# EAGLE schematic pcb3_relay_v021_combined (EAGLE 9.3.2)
Switching done with 30 x G6K-2F-Y 2xDPDT relays + 2 x HC-595

## Sheet 1 of 5: Amplitude & Frequency Detectors
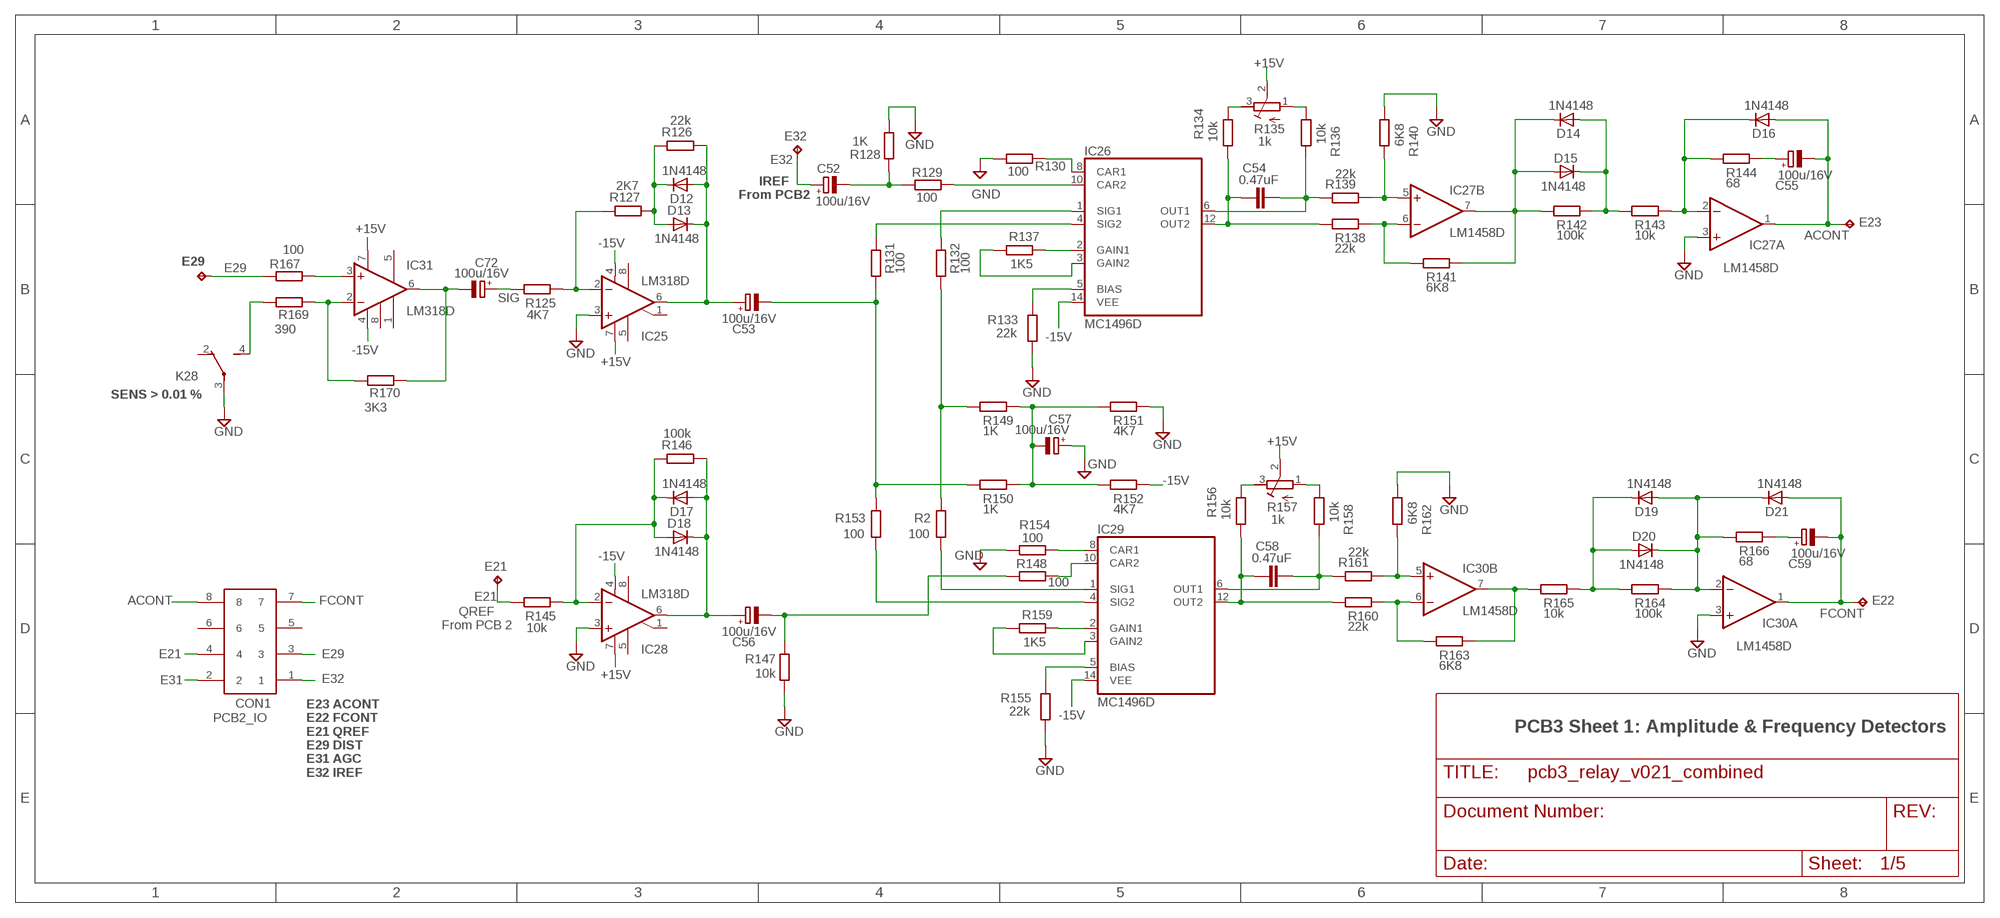
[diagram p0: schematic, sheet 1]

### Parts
C52  100u/16V  CPOL-EUUD-6,3X8,8  [UD-6,3X5,8_NICHICON]
C53  100u/16V  CPOL-EUUD-6,3X8,8  [UD-6,3X5,8_NICHICON]
C54  0.47uF  C-EUC1206  [C1206]
C55  100u/16V  CPOL-EUUD-6,3X8,8  [UD-6,3X5,8_NICHICON]
C56  100u/16V  CPOL-EUUD-6,3X8,8  [UD-6,3X5,8_NICHICON]
C57  100u/16V  CPOL-EUUD-6,3X8,8  [UD-6,3X5,8_NICHICON]
C58  0.47uF  C-EUC1206  [C1206]
C59  100u/16V  CPOL-EUUD-6,3X8,8  [UD-6,3X5,8_NICHICON]
C72  100u/16V  CPOL-EUUD-6,3X8,8  [UD-6,3X5,8_NICHICON]
CON1  PCB2_IO  61200821621  [61200821621]
D12  1N4148  D-SOD-80  [SOD80]
D13  1N4148  D-SOD-80  [SOD80]
D14  1N4148  D-SOD-80  [SOD80]
D15  1N4148  D-SOD-80  [SOD80]
D16  1N4148  D-SOD-80  [SOD80]
D17  1N4148  D-SOD-80  [SOD80]
D18  1N4148  D-SOD-80  [SOD80]
D19  1N4148  D-SOD-80  [SOD80]
D20  1N4148  D-SOD-80  [SOD80]
D21  1N4148  D-SOD-80  [SOD80]
E21  TPPAD1-13Y  [P1-13Y]
E22  TPPAD1-13Y  [P1-13Y]
E23  TPPAD1-13Y  [P1-13Y]
E29  TPPAD1-13Y  [P1-13Y]
E32  TPPAD1-13Y  [P1-13Y]
IC25  LM318D  [SO08]
IC26  MC1496D  [SOIC-14]
IC27  LM1458D  [SO08]
IC28  LM318D  [SO08]
IC29  MC1496D  [SOIC-14]
IC30  LM1458D  [SO08]
IC31  LM318D  [SOIC8]
K28  G6K-2F-Y  [G6K-2F-Y]
R2  100  R-EU_R1206  [R1206]
R125  4K7  R-EU_R1206  [R1206]
R126  22k  R-EU_R1206  [R1206]
R127  2K7  R-EU_R1206  [R1206]
R128  1K  R-EU_R1206  [R1206]
R129  100  R-EU_R1206  [R1206]
R130  100  R-EU_R1206  [R1206]
R131  100  R-EU_R1206  [R1206]
R132  100  R-EU_R1206  [R1206]
R133  22k  R-EU_R1206  [R1206]
R134  10k  R-EU_R1206  [R1206]
R135  1k  R-TRIMM3296W  [RTRIM3296W]
R136  10k  R-EU_R1206  [R1206]
R137  1K5  R-EU_R1206  [R1206]
R138  22k  R-EU_R1206  [R1206]
R139  22k  R-EU_R1206  [R1206]
R140  6K8  R-EU_R1206  [R1206]
R141  6K8  R-EU_R1206  [R1206]
R142  100k  R-EU_R1206  [R1206]
R143  10k  R-EU_R1206  [R1206]
R144  68  R-EU_R1206  [R1206]
R145  10k  R-EU_R1206  [R1206]
R146  100k  R-EU_R1206  [R1206]
R147  10k  R-EU_R1206  [R1206]
R148  100  R-EU_R1206  [R1206]
R149  1K  R-EU_R1206  [R1206]
R150  1K  R-EU_R1206  [R1206]
R151  4K7  R-EU_R1206  [R1206]
R152  4K7  R-EU_R1206  [R1206]
R153  100  R-EU_R1206  [R1206]
R154  100  R-EU_R1206  [R1206]
R155  22k  R-EU_R1206  [R1206]
R156  10k  R-EU_R1206  [R1206]
R157  1k  R-TRIMM3296W  [RTRIM3296W]
R158  10k  R-EU_R1206  [R1206]
R159  1K5  R-EU_R1206  [R1206]
R160  22k  R-EU_R1206  [R1206]
R161  22k  R-EU_R1206  [R1206]
R162  6K8  R-EU_R1206  [R1206]
R163  6K8  R-EU_R1206  [R1206]
R164  100k  R-EU_R1206  [R1206]
R165  10k  R-EU_R1206  [R1206]
R166  68  R-EU_R1206  [R1206]
R167  100  R-EU_R1206  [R1206]
R169  390  R-EU_R1206  [R1206]
R170  3K3  R-EU_R1206  [R1206]

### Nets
+15V: IC25.7(V+) IC28.7(V+) IC31.7(V+) R135.2(S) R157.2(S) ; also sheet 2,4,5
-15V: IC25.4(V-) IC26.14(VEE) IC28.4(V-) IC29.14(VEE) IC31.4(V-) R152.1 ; also sheet 2,4,5
ACONT: C55.- CON1.8 D16.2(A) E23.TP IC27.1(A:OUT)
E21: CON1.4 E21.TP R145.2
E29: CON1.3 E29.TP R167.1 ; also sheet 4
E31: CON1.2 ; also sheet 2
E32: C52.+ CON1.1 E32.TP
FCONT: C59.- CON1.7 D21.2(A) E22.TP IC30.1(A:OUT) ; also sheet 2
GND: C57.+ IC25.3(+IN) IC27.3(A:+IN) IC28.3(+IN) IC30.3(A:+IN) K28.3(2:P) R128.2 R130.2 R133.2 R140.2 R147.2 R151.1 R154.2 R155.2 R162.2 ; also sheet 2,3,4,5
N$1: IC26.8(CAR1) R130.1
N$17: IC25.2(-IN) R125.1 R127.1
N$22: D12.1(C) D13.2(A) R126.1 R127.2
N$24: C53.+ D12.2(A) D13.1(C) IC25.6(OUT) R126.2
N$27: D17.1(C) D18.2(A) IC28.2(-IN) R145.1 R146.1
N$28: C56.- R147.1 R148.2
N$29: C56.+ D17.2(A) D18.1(C) IC28.6(OUT) R146.2
N$30: IC26.3(GAIN2) R137.2
N$31: IC26.10(CAR2) R129.1
N$35: IC29.2(GAIN1) R159.1
N$36: R134.1 R135.3(E)
N$37: IC26.2(GAIN1) R137.1
N$38: IC26.5(BIAS) R133.1
N$39: IC29.5(BIAS) R155.1
N$40: IC29.8(CAR1) R154.1
N$41: IC26.4(SIG2) R131.1
N$42: IC26.1(SIG1) R132.1
N$43: C52.- R128.1 R129.2
N$44: C58.1 IC29.12(OUT2) R156.2 R160.2
N$45: C54.2 IC26.6(OUT1) R136.1 R139.1
N$46: C54.1 IC26.12(OUT2) R134.2 R138.2
N$47: IC27.5(B:+IN) R139.2 R140.1
N$48: IC27.6(B:-IN) R138.1 R141.2
N$49: IC29.10(CAR2) R148.1
N$50: D14.1(C) D15.2(A) IC27.7(B:OUT) R141.1 R142.2
N$51: D14.2(A) D15.1(C) R142.1 R143.2
N$52: D16.1(C) IC27.2(A:-IN) R143.1 R144.2
N$53: C55.+ R144.1
N$54: C53.- R131.2 R150.2 R153.1
N$55: R135.1(A) R136.2
N$56: IC29.4(SIG2) R153.2
N$57: IC29.3(GAIN2) R159.2
N$58: R156.1 R157.3(E)
N$59: R157.1(A) R158.2
N$60: C58.2 IC29.6(OUT1) R158.1 R161.1
N$61: IC30.5(B:+IN) R161.2 R162.1
N$62: IC30.6(B:-IN) R160.1 R163.2
N$63: D19.1(C) D20.2(A) R164.2 R165.1
N$64: D19.2(A) D20.1(C) D21.1(C) IC30.2(A:-IN) R164.1 R166.2
N$65: C72.- IC31.6(OUT) R170.1
N$66: C59.+ R166.1
N$67: IC29.1(SIG1) R2.2
N$68: R2.1 R132.2 R149.2
N$69: C57.- R149.1 R150.1 R151.2 R152.2
N$70: IC30.7(B:OUT) R163.1 R165.2
N$71: IC31.3(+IN) R167.2
N$72: K28.4(2:S) R169.2
N$73: IC31.2(-IN) R169.1 R170.2
SIG: C72.+ R125.2
Unconnected: CON1.5 CON1.6 IC25.1(ON/CMP) IC25.5(ON) IC25.8(CMP) IC28.1(ON/CMP) IC28.5(ON) IC28.8(CMP) IC31.1(BAL1) IC31.5(BAL2) IC31.8(COMP) K28.2(2:O)

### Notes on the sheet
- IREF
  From PCB2
- SENS > 0.01 %
- QREF
  From PCB 2
- PCB3 Sheet 1: Amplitude & Frequency Detectors
- E23 ACONT
  E22 FCONT
  E21 QREF
  E29 DIST
  E31 AGC
  E32 IREF

## Sheet 2 of 5: Meter + LEDs
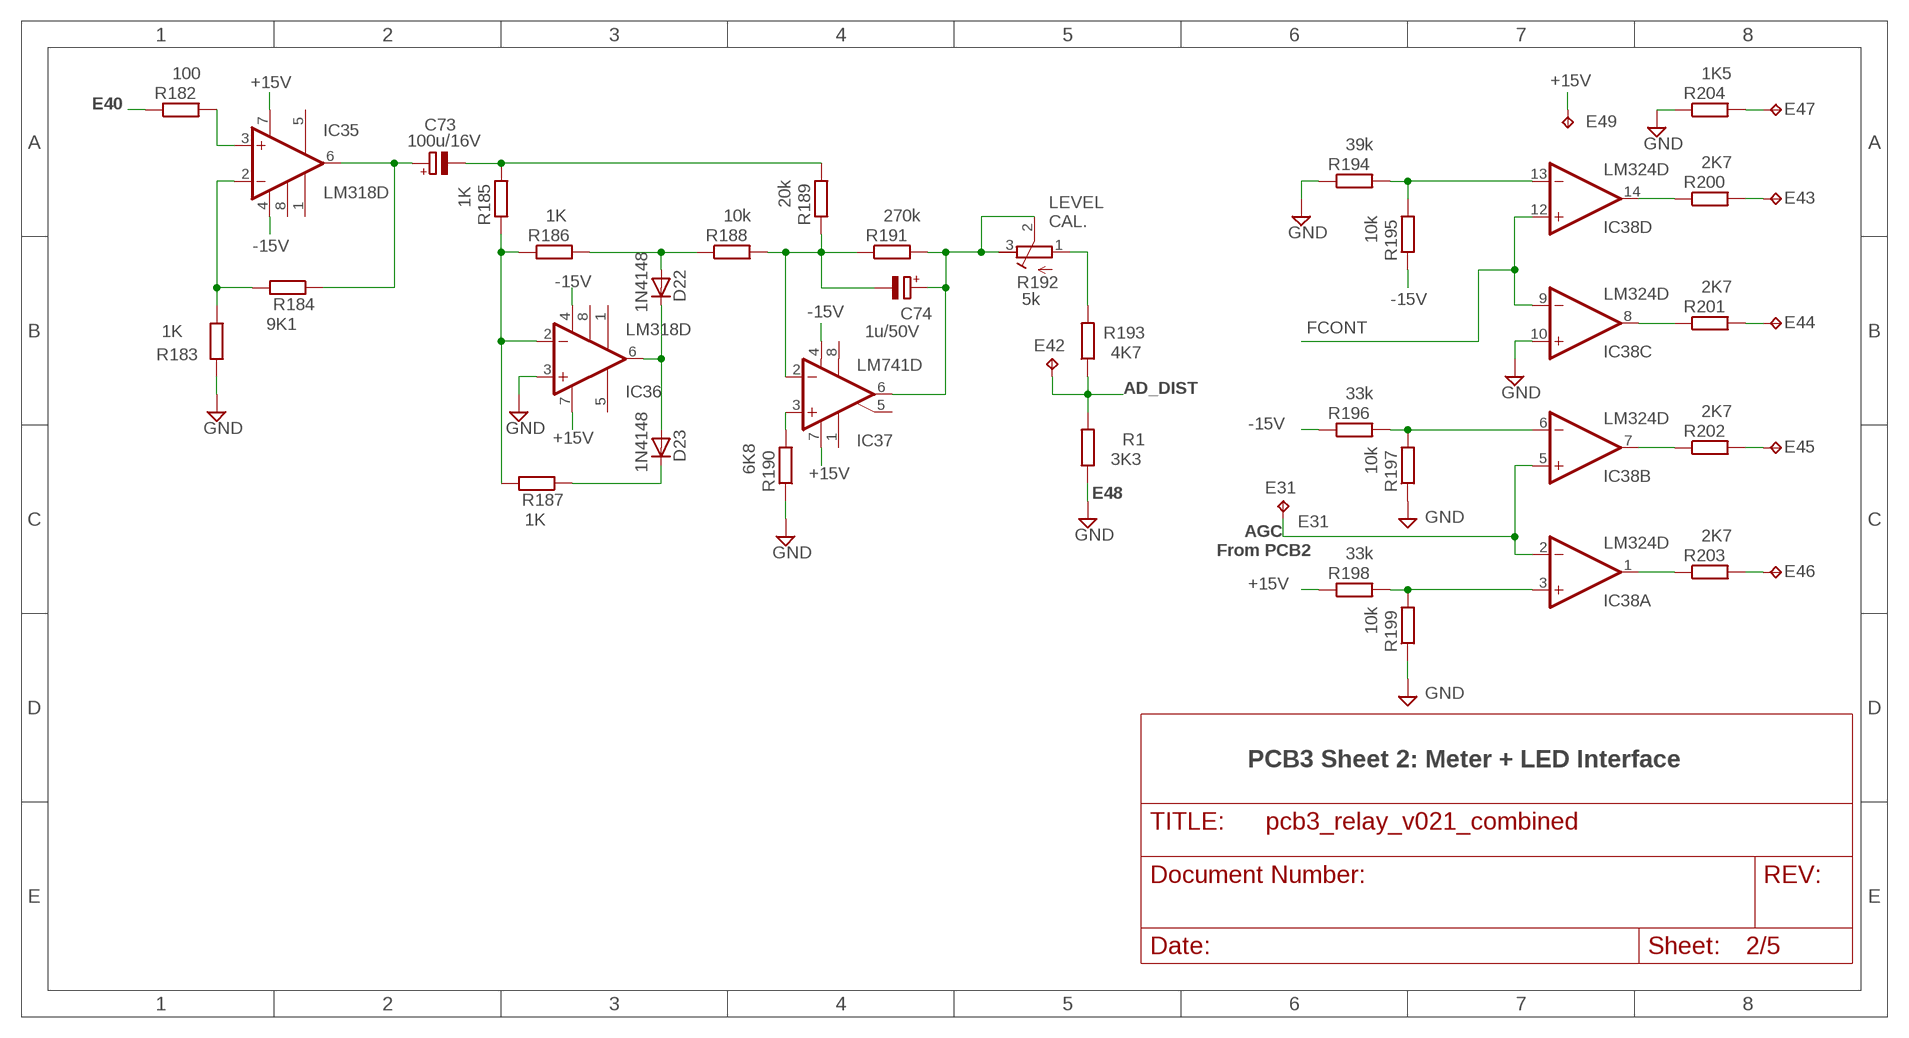
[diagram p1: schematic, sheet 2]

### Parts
C73  100u/16V  CPOL-EUUD-6,3X8,8  [UD-6,3X5,8_NICHICON]
C74  1u/50V  CPOL-EUUD-4X5,8  [UD-4X5,8_NICHICON]
D22  1N4148  D-SOD-80  [SOD80]
D23  1N4148  D-SOD-80  [SOD80]
E31  TPPAD1-13Y  [P1-13Y]
E42  TPPAD1-13Y  [P1-13Y]
E43  TPPAD1-13Y  [P1-13Y]
E44  TPPAD1-13Y  [P1-13Y]
E45  TPPAD1-13Y  [P1-13Y]
E46  TPPAD1-13Y  [P1-13Y]
E47  TPPAD1-13Y  [P1-13Y]
E49  TPPAD1-13Y  [P1-13Y]
IC35  LM318D  [SOIC8]
IC36  LM318D  [SOIC8]
IC37  LM741D  [SO08]
IC38  LM324D  [SO14]
R1  3K3  R-EU_R1206  [R1206]
R182  100  R-EU_R1206  [R1206]
R183  1K  R-EU_R1206  [R1206]
R184  9K1  R-EU_R1206  [R1206]
R185  1K  R-EU_R1206  [R1206]
R186  1K  R-EU_R1206  [R1206]
R187  1K  R-EU_R1206  [R1206]
R188  10k  R-EU_R1206  [R1206]
R189  20k  R-EU_R1206  [R1206]
R190  6K8  R-EU_R1206  [R1206]
R191  270k  R-EU_R1206  [R1206]
R192  5k  R-TRIMM3296W  [RTRIM3296W]
R193  4K7  R-EU_R1206  [R1206]
R194  39k  R-EU_R1206  [R1206]
R195  10k  R-EU_R1206  [R1206]
R196  33k  R-EU_R1206  [R1206]
R197  10k  R-EU_R1206  [R1206]
R198  33k  R-EU_R1206  [R1206]
R199  10k  R-EU_R1206  [R1206]
R200  2K7  R-EU_R1206  [R1206]
R201  2K7  R-EU_R1206  [R1206]
R202  2K7  R-EU_R1206  [R1206]
R203  2K7  R-EU_R1206  [R1206]
R204  1K5  R-EU_R1206  [R1206]

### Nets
+15V: E49.TP IC35.7(V+) IC36.7(V+) IC37.7(V+) R198.1 ; also sheet 1,4,5
-15V: IC35.4(V-) IC36.4(V-) IC37.4(V-) R195.1 R196.1 ; also sheet 1,4,5
AD_DIST: E42.TP R1.2 R193.1 ; also sheet 3
E31: E31.TP IC38.2(A:-IN) IC38.5(B:+IN) ; also sheet 1
E40: R182.1 ; also sheet 4
E43: E43.TP R200.2
E44: E44.TP R201.2
E45: E45.TP R202.2
E46: E46.TP R203.2
FCONT: IC38.9(C:-IN) IC38.12(D:+IN) ; also sheet 1
GND: IC36.3(+IN) IC38.10(C:+IN) R1.1 R183.2 R190.1 R194.1 R197.1 R199.1 R204.1 ; also sheet 1,3,4,5
N$2: R192.1(A) R193.2
N$3: IC37.3(+IN) R190.2
N$4: IC36.2(-IN) R185.1 R186.1 R187.2
N$5: D23.1(C) R187.1
N$6: D22.1(C) D23.2(A) IC36.6(OUT)
N$7: D22.2(A) R186.2 R188.1
N$8: C74.- IC37.2(-IN) R188.2 R189.1 R191.1
N$9: C74.+ IC37.6(OUT) R191.2 R192.2(S) R192.3(E)
N$10: C73.- R185.2 R189.2
N$11: IC38.13(D:-IN) R194.2 R195.2
N$12: IC38.3(A:+IN) R198.2 R199.2
N$13: IC38.6(B:-IN) R196.2 R197.2
N$14: IC38.1(A:OUT) R203.1
N$15: E47.TP R204.2
N$16: IC35.2(-IN) R183.1 R184.2
N$18: IC38.7(B:OUT) R202.1
N$19: IC38.8(C:OUT) R201.1
N$25: IC38.14(D:OUT) R200.1
N$81: IC35.3(+IN) R182.2
N$84: C73.+ IC35.6(OUT) R184.1
Unconnected: IC35.1(BAL1) IC35.5(BAL2) IC35.8(COMP) IC36.1(BAL1) IC36.5(BAL2) IC36.8(COMP) IC37.1(ON1) IC37.5(ON2) IC37.8(OPT)

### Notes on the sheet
- LEVEL
  CAL.
- E48
- AGC
  From PCB2
- PCB3 Sheet 2: Meter + LED Interface

## Sheet 3 of 5: Relays + Digital
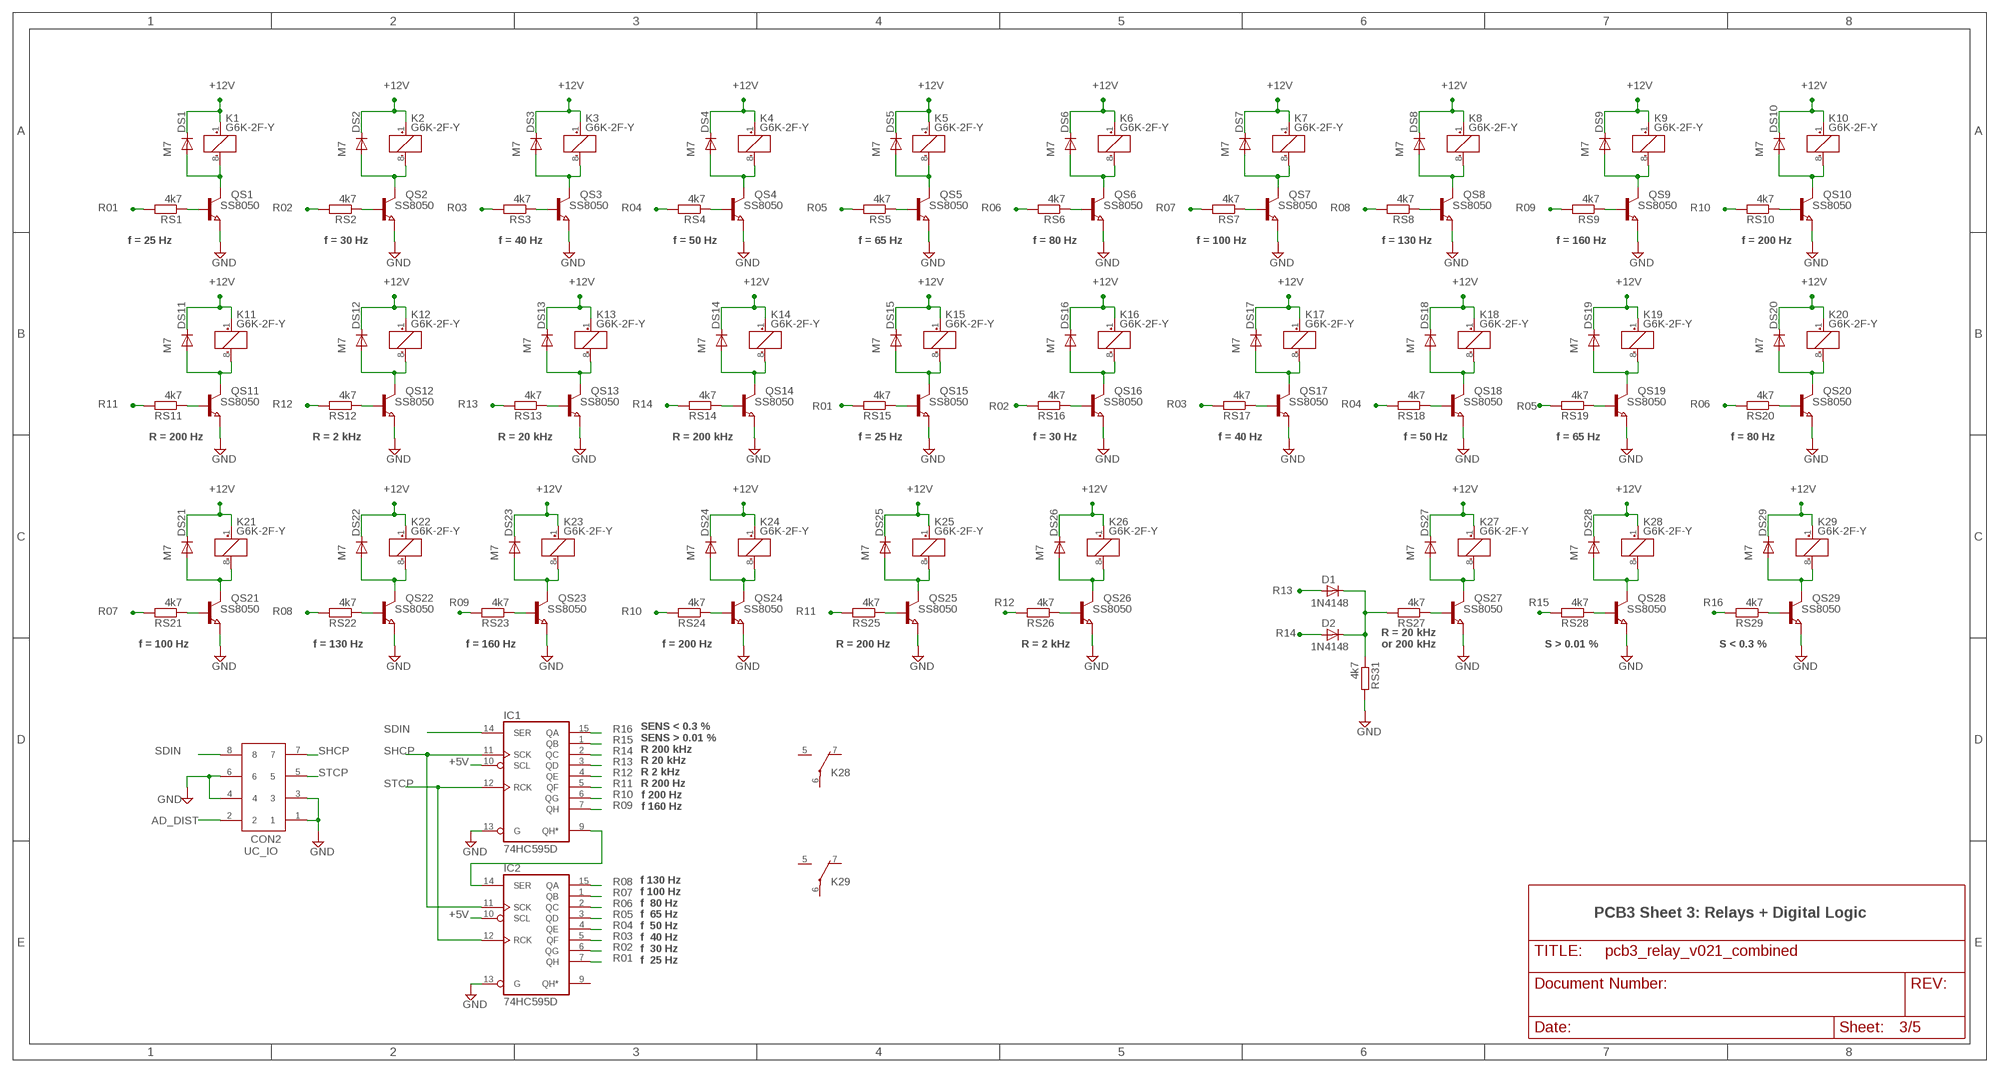
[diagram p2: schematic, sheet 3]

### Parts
CON2  UC_IO  61200821621  [61200821621]
D1  1N4148  D-SOD-80  [SOD80]
D2  1N4148  D-SOD-80  [SOD80]
DS1  M7  DIODE-DO214AC  [DO214AC]
DS2  M7  DIODE-DO214AC  [DO214AC]
DS3  M7  DIODE-DO214AC  [DO214AC]
DS4  M7  DIODE-DO214AC  [DO214AC]
DS5  M7  DIODE-DO214AC  [DO214AC]
DS6  M7  DIODE-DO214AC  [DO214AC]
DS7  M7  DIODE-DO214AC  [DO214AC]
DS8  M7  DIODE-DO214AC  [DO214AC]
DS9  M7  DIODE-DO214AC  [DO214AC]
DS10  M7  DIODE-DO214AC  [DO214AC]
DS11  M7  DIODE-DO214AC  [DO214AC]
DS12  M7  DIODE-DO214AC  [DO214AC]
DS13  M7  DIODE-DO214AC  [DO214AC]
DS14  M7  DIODE-DO214AC  [DO214AC]
DS15  M7  DIODE-DO214AC  [DO214AC]
DS16  M7  DIODE-DO214AC  [DO214AC]
DS17  M7  DIODE-DO214AC  [DO214AC]
DS18  M7  DIODE-DO214AC  [DO214AC]
DS19  M7  DIODE-DO214AC  [DO214AC]
DS20  M7  DIODE-DO214AC  [DO214AC]
DS21  M7  DIODE-DO214AC  [DO214AC]
DS22  M7  DIODE-DO214AC  [DO214AC]
DS23  M7  DIODE-DO214AC  [DO214AC]
DS24  M7  DIODE-DO214AC  [DO214AC]
DS25  M7  DIODE-DO214AC  [DO214AC]
DS26  M7  DIODE-DO214AC  [DO214AC]
DS27  M7  DIODE-DO214AC  [DO214AC]
DS28  M7  DIODE-DO214AC  [DO214AC]
DS29  M7  DIODE-DO214AC  [DO214AC]
IC1  74HC595D  [SO16]
IC2  74HC595D  [SO16]
K1  G6K-2F-Y  [G6K-2F-Y]
K2  G6K-2F-Y  [G6K-2F-Y]
K3  G6K-2F-Y  [G6K-2F-Y]
K4  G6K-2F-Y  [G6K-2F-Y]
K5  G6K-2F-Y  [G6K-2F-Y]
K6  G6K-2F-Y  [G6K-2F-Y]
K7  G6K-2F-Y  [G6K-2F-Y]
K8  G6K-2F-Y  [G6K-2F-Y]
K9  G6K-2F-Y  [G6K-2F-Y]
K10  G6K-2F-Y  [G6K-2F-Y]
K11  G6K-2F-Y  [G6K-2F-Y]
K12  G6K-2F-Y  [G6K-2F-Y]
K13  G6K-2F-Y  [G6K-2F-Y]
K14  G6K-2F-Y  [G6K-2F-Y]
K15  G6K-2F-Y  [G6K-2F-Y]
K16  G6K-2F-Y  [G6K-2F-Y]
K17  G6K-2F-Y  [G6K-2F-Y]
K18  G6K-2F-Y  [G6K-2F-Y]
K19  G6K-2F-Y  [G6K-2F-Y]
K20  G6K-2F-Y  [G6K-2F-Y]
K21  G6K-2F-Y  [G6K-2F-Y]
K22  G6K-2F-Y  [G6K-2F-Y]
K23  G6K-2F-Y  [G6K-2F-Y]
K24  G6K-2F-Y  [G6K-2F-Y]
K25  G6K-2F-Y  [G6K-2F-Y]
K26  G6K-2F-Y  [G6K-2F-Y]
K27  G6K-2F-Y  [G6K-2F-Y]
K29  G6K-2F-Y  [G6K-2F-Y]
QS1  SS8050  NPN-TRANSISTOR_SOT23  [SOT23]
QS2  SS8050  NPN-TRANSISTOR_SOT23  [SOT23]
QS3  SS8050  NPN-TRANSISTOR_SOT23  [SOT23]
QS4  SS8050  NPN-TRANSISTOR_SOT23  [SOT23]
QS5  SS8050  NPN-TRANSISTOR_SOT23  [SOT23]
QS6  SS8050  NPN-TRANSISTOR_SOT23  [SOT23]
QS7  SS8050  NPN-TRANSISTOR_SOT23  [SOT23]
QS8  SS8050  NPN-TRANSISTOR_SOT23  [SOT23]
QS9  SS8050  NPN-TRANSISTOR_SOT23  [SOT23]
QS10  SS8050  NPN-TRANSISTOR_SOT23  [SOT23]
QS11  SS8050  NPN-TRANSISTOR_SOT23  [SOT23]
QS12  SS8050  NPN-TRANSISTOR_SOT23  [SOT23]
QS13  SS8050  NPN-TRANSISTOR_SOT23  [SOT23]
QS14  SS8050  NPN-TRANSISTOR_SOT23  [SOT23]
QS15  SS8050  NPN-TRANSISTOR_SOT23  [SOT23]
QS16  SS8050  NPN-TRANSISTOR_SOT23  [SOT23]
QS17  SS8050  NPN-TRANSISTOR_SOT23  [SOT23]
QS18  SS8050  NPN-TRANSISTOR_SOT23  [SOT23]
QS19  SS8050  NPN-TRANSISTOR_SOT23  [SOT23]
QS20  SS8050  NPN-TRANSISTOR_SOT23  [SOT23]
QS21  SS8050  NPN-TRANSISTOR_SOT23  [SOT23]
QS22  SS8050  NPN-TRANSISTOR_SOT23  [SOT23]
QS23  SS8050  NPN-TRANSISTOR_SOT23  [SOT23]
QS24  SS8050  NPN-TRANSISTOR_SOT23  [SOT23]
QS25  SS8050  NPN-TRANSISTOR_SOT23  [SOT23]
QS26  SS8050  NPN-TRANSISTOR_SOT23  [SOT23]
QS27  SS8050  NPN-TRANSISTOR_SOT23  [SOT23]
QS28  SS8050  NPN-TRANSISTOR_SOT23  [SOT23]
QS29  SS8050  NPN-TRANSISTOR_SOT23  [SOT23]
RS1  4k7  R-EU_M1206  [M1206]
RS2  4k7  R-EU_M1206  [M1206]
RS3  4k7  R-EU_M1206  [M1206]
RS4  4k7  R-EU_M1206  [M1206]
RS5  4k7  R-EU_M1206  [M1206]
RS6  4k7  R-EU_M1206  [M1206]
RS7  4k7  R-EU_M1206  [M1206]
RS8  4k7  R-EU_M1206  [M1206]
RS9  4k7  R-EU_M1206  [M1206]
RS10  4k7  R-EU_M1206  [M1206]
RS11  4k7  R-EU_M1206  [M1206]
RS12  4k7  R-EU_M1206  [M1206]
RS13  4k7  R-EU_M1206  [M1206]
RS14  4k7  R-EU_M1206  [M1206]
RS15  4k7  R-EU_M1206  [M1206]
RS16  4k7  R-EU_M1206  [M1206]
RS17  4k7  R-EU_M1206  [M1206]
RS18  4k7  R-EU_M1206  [M1206]
RS19  4k7  R-EU_M1206  [M1206]
RS20  4k7  R-EU_M1206  [M1206]
RS21  4k7  R-EU_M1206  [M1206]
RS22  4k7  R-EU_M1206  [M1206]
RS23  4k7  R-EU_M1206  [M1206]
RS24  4k7  R-EU_M1206  [M1206]
RS25  4k7  R-EU_M1206  [M1206]
RS26  4k7  R-EU_M1206  [M1206]
RS27  4k7  R-EU_M1206  [M1206]
RS28  4k7  R-EU_M1206  [M1206]
RS29  4k7  R-EU_M1206  [M1206]
RS31  4k7  R-EU_M1206  [M1206]

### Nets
+5V: IC1.10(SCL) IC2.10(SCL) ; also sheet 5
+12V: DS1.C DS2.C DS3.C DS4.C DS5.C DS6.C DS7.C DS8.C DS9.C DS10.C DS11.C DS12.C DS13.C DS14.C DS15.C DS16.C DS17.C DS18.C DS19.C DS20.C DS21.C DS22.C DS23.C DS24.C DS25.C DS26.C DS27.C DS28.C DS29.C K1.1(1:+) K2.1(1:+) K3.1(1:+) K4.1(1:+) K5.1(1:+) K6.1(1:+) K7.1(1:+) K8.1(1:+) K9.1(1:+) K10.1(1:+) K11.1(1:+) K12.1(1:+) K13.1(1:+) K14.1(1:+) K15.1(1:+) K16.1(1:+) K17.1(1:+) K18.1(1:+) K19.1(1:+) K20.1(1:+) K21.1(1:+) K22.1(1:+) K23.1(1:+) K24.1(1:+) K25.1(1:+) K26.1(1:+) K27.1(1:+) K28.1(1:+) K29.1(1:+) ; also sheet 5
AD_DIST: CON2.2 ; also sheet 2
GND: CON2.1 CON2.3 CON2.4 CON2.6 IC1.13(G) IC2.13(G) QS1.2(E) QS2.2(E) QS3.2(E) QS4.2(E) QS5.2(E) QS6.2(E) QS7.2(E) QS8.2(E) QS9.2(E) QS10.2(E) QS11.2(E) QS12.2(E) QS13.2(E) QS14.2(E) QS15.2(E) QS16.2(E) QS17.2(E) QS18.2(E) QS19.2(E) QS20.2(E) QS21.2(E) QS22.2(E) QS23.2(E) QS24.2(E) QS25.2(E) QS26.2(E) QS27.2(E) QS28.2(E) QS29.2(E) RS31.2 ; also sheet 1,2,4,5
N$74: D1.1(C) D2.1(C) RS27.2 RS31.1
N$101: QS1.1(B) RS1.1
N$102: DS1.A K1.8(1:-) QS1.3(C)
N$103: QS2.1(B) RS2.1
N$104: DS2.A K2.8(1:-) QS2.3(C)
N$105: QS3.1(B) RS3.1
N$106: DS3.A K3.8(1:-) QS3.3(C)
N$107: QS4.1(B) RS4.1
N$108: DS4.A K4.8(1:-) QS4.3(C)
N$109: QS5.1(B) RS5.1
N$110: DS5.A K5.8(1:-) QS5.3(C)
N$111: QS6.1(B) RS6.1
N$112: DS6.A K6.8(1:-) QS6.3(C)
N$113: QS7.1(B) RS7.1
N$114: DS7.A K7.8(1:-) QS7.3(C)
N$115: QS8.1(B) RS8.1
N$116: DS8.A K8.8(1:-) QS8.3(C)
N$117: QS9.1(B) RS9.1
N$118: DS9.A K9.8(1:-) QS9.3(C)
N$119: QS10.1(B) RS10.1
N$120: DS10.A K10.8(1:-) QS10.3(C)
N$124: QS11.1(B) RS11.1
N$125: DS11.A K11.8(1:-) QS11.3(C)
N$126: QS12.1(B) RS12.1
N$127: DS12.A K12.8(1:-) QS12.3(C)
N$128: QS13.1(B) RS13.1
N$129: DS13.A K13.8(1:-) QS13.3(C)
N$130: QS14.1(B) RS14.1
N$131: DS14.A K14.8(1:-) QS14.3(C)
N$132: QS16.1(B) RS16.1
N$133: DS16.A K16.8(1:-) QS16.3(C)
N$134: QS17.1(B) RS17.1
N$135: DS17.A K17.8(1:-) QS17.3(C)
N$136: QS18.1(B) RS18.1
N$137: DS18.A K18.8(1:-) QS18.3(C)
N$138: QS23.1(B) RS23.1
N$139: DS23.A K23.8(1:-) QS23.3(C)
N$140: QS19.1(B) RS19.1
N$141: DS19.A K19.8(1:-) QS19.3(C)
N$142: QS20.1(B) RS20.1
N$143: DS20.A K20.8(1:-) QS20.3(C)
N$144: QS21.1(B) RS21.1
N$145: DS21.A K21.8(1:-) QS21.3(C)
N$146: QS22.1(B) RS22.1
N$147: DS22.A K22.8(1:-) QS22.3(C)
N$148: QS15.1(B) RS15.1
N$149: DS15.A K15.8(1:-) QS15.3(C)
N$151: IC1.9(QH*) IC2.14(SER)
N$183: QS27.1(B) RS27.1
N$184: DS27.A K27.8(1:-) QS27.3(C)
N$185: QS24.1(B) RS24.1
N$186: DS24.A K24.8(1:-) QS24.3(C)
N$187: QS25.1(B) RS25.1
N$188: DS25.A K25.8(1:-) QS25.3(C)
N$189: QS26.1(B) RS26.1
N$190: DS26.A K26.8(1:-) QS26.3(C)
N$193: QS28.1(B) RS28.1
N$194: DS28.A K28.8(1:-) QS28.3(C)
N$195: QS29.1(B) RS29.1
N$196: DS29.A K29.8(1:-) QS29.3(C)
R01: IC2.7(QH) RS1.2 RS15.2
R02: IC2.6(QG) RS2.2 RS16.2
R03: IC2.5(QF) RS3.2 RS17.2
R04: IC2.4(QE) RS4.2 RS18.2
R05: IC2.3(QD) RS5.2 RS19.2
R06: IC2.2(QC) RS6.2 RS20.2
R07: IC2.1(QB) RS7.2 RS21.2
R08: IC2.15(QA) RS8.2 RS22.2
R09: IC1.7(QH) RS9.2 RS23.2
R10: IC1.6(QG) RS10.2 RS24.2
R11: IC1.5(QF) RS11.2 RS25.2
R12: IC1.4(QE) RS12.2 RS26.2
R13: D1.2(A) IC1.3(QD) RS13.2
R14: D2.2(A) IC1.2(QC) RS14.2
R15: IC1.1(QB) RS28.2
R16: IC1.15(QA) RS29.2
SDIN: CON2.8 IC1.14(SER)
SHCP: CON2.7 IC1.11(SCK) IC2.11(SCK)
STCP: CON2.5 IC1.12(RCK) IC2.12(RCK)
Unconnected: IC2.9(QH*) K28.5(3:S) K28.6(3:P) K28.7(3:O) K29.5(3:S) K29.6(3:P) K29.7(3:O)

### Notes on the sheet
- f = 25 Hz | f = 30 Hz | f = 40 Hz | f = 50 Hz | f = 65 Hz | f = 80 Hz | f = 100 Hz | f = 130 Hz | f = 160 Hz | f = 200 Hz
- R = 200 Hz | R = 2 kHz | R = 20 kHz | R = 200 kHz | f = 25 Hz | f = 30 Hz | f = 40 Hz | f = 50 Hz | f = 65 Hz | f = 80 Hz
- f = 100 Hz | f = 130 Hz | f = 160 Hz | f = 200 Hz | R = 200 Hz | R = 2 kHz
- R = 20 kHz
  or 200 kHz
- S > 0.01 % | S < 0.3 %
- SENS < 0.3 %
  SENS > 0.01 %
  R 200 kHz
  R 20 kHz
  R 2 kHz
  R 200 Hz
  f 200 Hz
  f 160 Hz
- PCB3 Sheet 3: Relays + Digital Logic
- f 130 Hz
  f 100 Hz
  f  80 Hz
  f  65 Hz
  f  50 Hz
  f  40 Hz
  f  30 Hz
  f  25 Hz

## Sheet 4 of 5: Filter Circuit
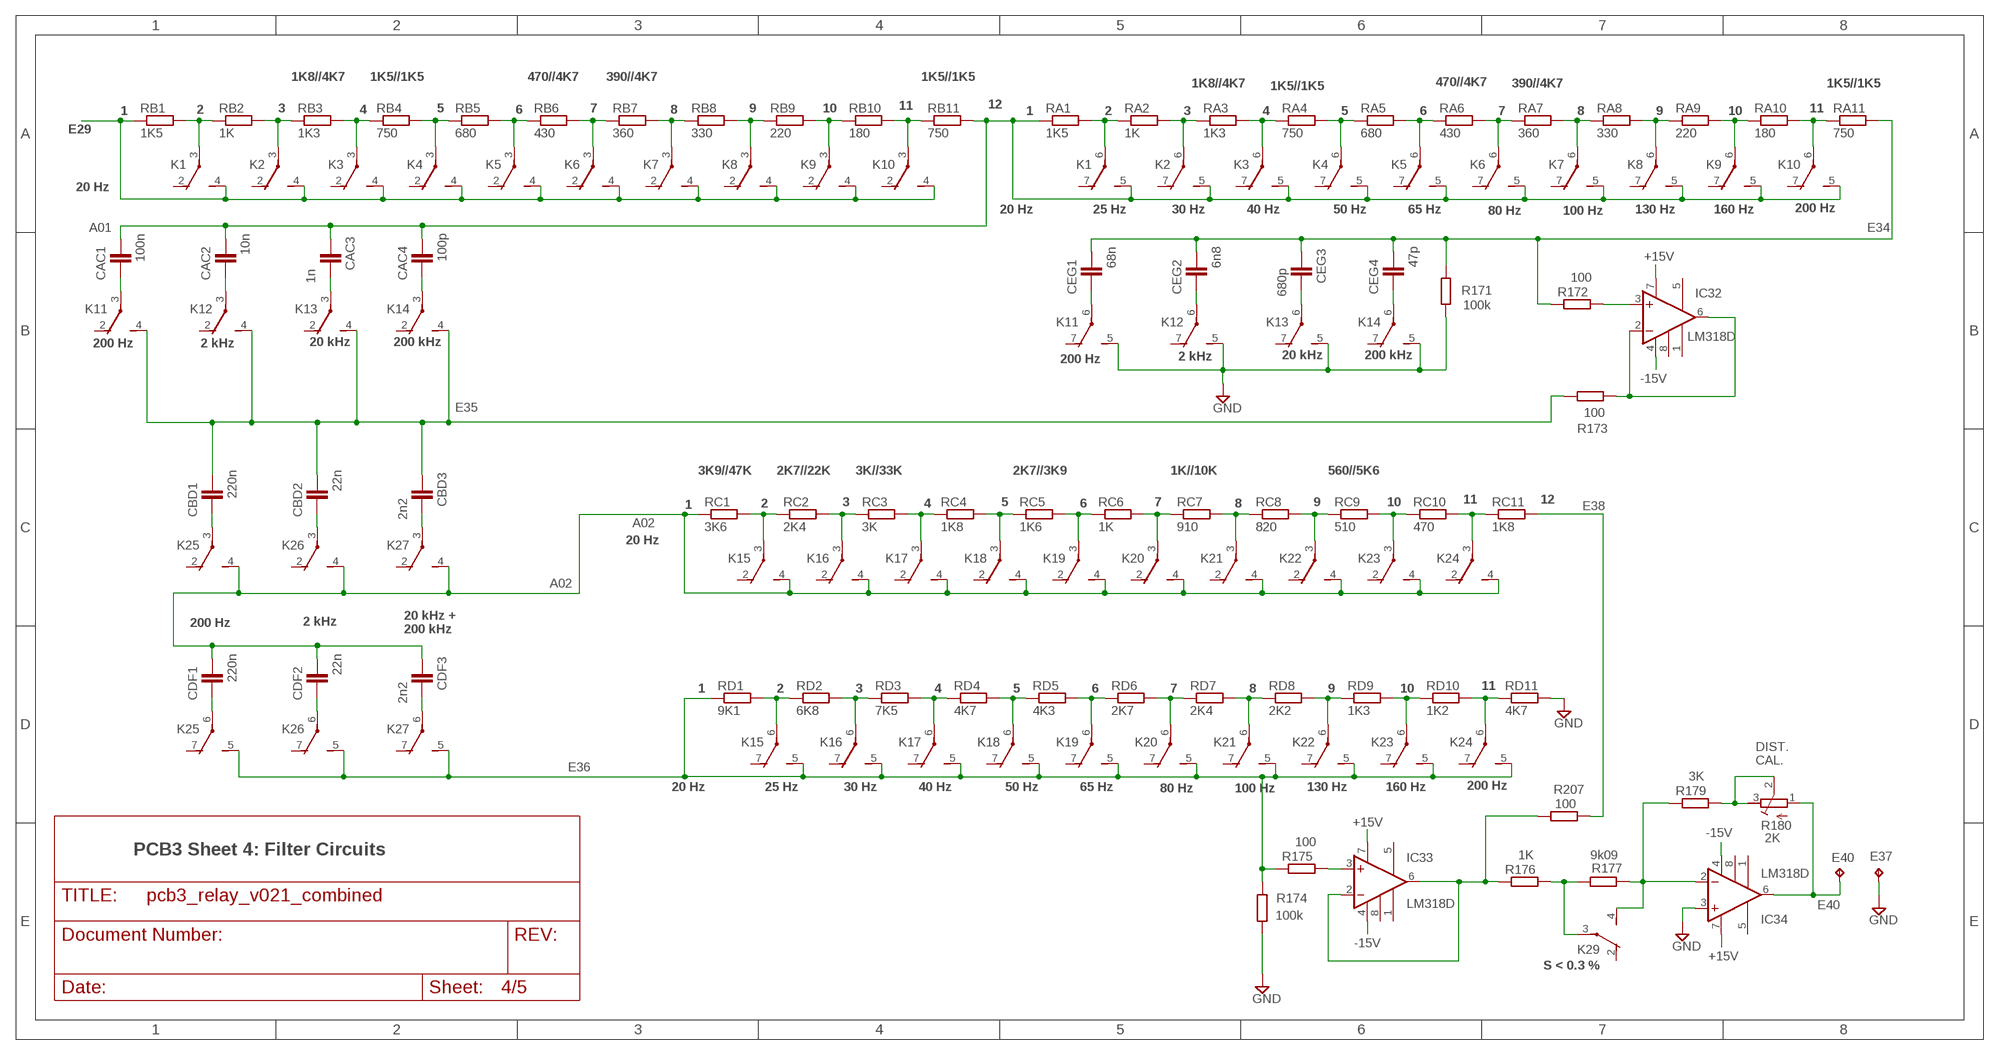
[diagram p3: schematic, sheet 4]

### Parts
CAC1  100n  C-EUC1206  [C1206]
CAC2  10n  C-EUC1206  [C1206]
CAC3  1n  C-EUC1206  [C1206]
CAC4  100p  C-EUC1206  [C1206]
CBD1  220n  C-EUC1206  [C1206]
CBD2  22n  C-EUC1206  [C1206]
CBD3  2n2  C-EUC1206  [C1206]
CDF1  220n  C-EUC1206  [C1206]
CDF2  22n  C-EUC1206  [C1206]
CDF3  2n2  C-EUC1206  [C1206]
CEG1  68n  C-EUC1206  [C1206]
CEG2  6n8  C-EUC1206  [C1206]
CEG3  680p  C-EUC1206  [C1206]
CEG4  47p  C-EUC1206  [C1206]
E37  TPPAD1-13Y  [P1-13Y]
E40  TPPAD1-13Y  [P1-13Y]
IC32  LM318D  [SOIC8]
IC33  LM318D  [SOIC8]
IC34  LM318D  [SOIC8]
R171  100k  R-EU_R1206  [R1206]
R172  100  R-EU_R1206  [R1206]
R173  100  R-EU_R1206  [R1206]
R174  100k  R-EU_R1206  [R1206]
R175  100  R-EU_R1206  [R1206]
R176  1K  R-EU_R1206  [R1206]
R177  9k09  R-EU_R1206  [R1206]
R179  3K  R-EU_R1206  [R1206]
R180  2K  R-TRIMM3296W  [RTRIM3296W]
R207  100  R-EU_R1206  [R1206]
RA1  1K5  R-EU_R1206  [R1206]
RA2  1K  R-EU_R1206  [R1206]
RA3  1K3  R-EU_R1206  [R1206]
RA4  750  R-EU_R1206  [R1206]
RA5  680  R-EU_R1206  [R1206]
RA6  430  R-EU_R1206  [R1206]
RA7  360  R-EU_R1206  [R1206]
RA8  330  R-EU_R1206  [R1206]
RA9  220  R-EU_R1206  [R1206]
RA10  180  R-EU_R1206  [R1206]
RA11  750  R-EU_R1206  [R1206]
RB1  1K5  R-EU_R1206  [R1206]
RB2  1K  R-EU_R1206  [R1206]
RB3  1K3  R-EU_R1206  [R1206]
RB4  750  R-EU_R1206  [R1206]
RB5  680  R-EU_R1206  [R1206]
RB6  430  R-EU_R1206  [R1206]
RB7  360  R-EU_R1206  [R1206]
RB8  330  R-EU_R1206  [R1206]
RB9  220  R-EU_R1206  [R1206]
RB10  180  R-EU_R1206  [R1206]
RB11  750  R-EU_R1206  [R1206]
RC1  3K6  R-EU_R1206  [R1206]
RC2  2K4  R-EU_R1206  [R1206]
RC3  3K  R-EU_R1206  [R1206]
RC4  1K8  R-EU_R1206  [R1206]
RC5  1K6  R-EU_R1206  [R1206]
RC6  1K  R-EU_R1206  [R1206]
RC7  910  R-EU_R1206  [R1206]
RC8  820  R-EU_R1206  [R1206]
RC9  510  R-EU_R1206  [R1206]
RC10  470  R-EU_R1206  [R1206]
RC11  1K8  R-EU_R1206  [R1206]
RD1  9K1  R-EU_R1206  [R1206]
RD2  6K8  R-EU_R1206  [R1206]
RD3  7K5  R-EU_R1206  [R1206]
RD4  4K7  R-EU_R1206  [R1206]
RD5  4K3  R-EU_R1206  [R1206]
RD6  2K7  R-EU_R1206  [R1206]
RD7  2K4  R-EU_R1206  [R1206]
RD8  2K2  R-EU_R1206  [R1206]
RD9  1K3  R-EU_R1206  [R1206]
RD10  1K2  R-EU_R1206  [R1206]
RD11  4K7  R-EU_R1206  [R1206]

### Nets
+15V: IC32.7(V+) IC33.7(V+) IC34.7(V+) ; also sheet 1,2,5
-15V: IC32.4(V-) IC33.4(V-) IC34.4(V-) ; also sheet 1,2,5
A01: CAC1.2 CAC2.2 CAC3.1 CAC4.2 K1.5(3:S) K2.5(3:S) K3.5(3:S) K4.5(3:S) K5.5(3:S) K6.5(3:S) K7.5(3:S) K8.5(3:S) K9.5(3:S) K10.5(3:S) RA1.1 RB11.2
A02: CDF1.2 CDF2.2 CDF3.1 K15.4(2:S) K16.4(2:S) K17.4(2:S) K18.4(2:S) K19.4(2:S) K20.4(2:S) K21.4(2:S) K22.4(2:S) K23.4(2:S) K24.4(2:S) K25.4(2:S) K26.4(2:S) K27.4(2:S) RC1.1
E29: K1.4(2:S) K2.4(2:S) K3.4(2:S) K4.4(2:S) K5.4(2:S) K6.4(2:S) K7.4(2:S) K8.4(2:S) K9.4(2:S) K10.4(2:S) RB1.1 ; also sheet 1
E34: CEG1.2 CEG2.2 CEG3.1 CEG4.2 R171.2 R172.1 RA11.2
E35: CBD1.2 CBD2.2 CBD3.1 K11.4(2:S) K12.4(2:S) K13.4(2:S) K14.4(2:S) R173.2
E36: K15.5(3:S) K16.5(3:S) K17.5(3:S) K18.5(3:S) K19.5(3:S) K20.5(3:S) K21.5(3:S) K22.5(3:S) K23.5(3:S) K24.5(3:S) K25.5(3:S) K26.5(3:S) K27.5(3:S) R174.2 R175.1 RD1.1
E38: R207.1 RC11.2
E40: E40.TP IC34.6(OUT) R180.1(A) ; also sheet 2
GND: E37.TP IC34.3(+IN) K11.5(3:S) K12.5(3:S) K13.5(3:S) K14.5(3:S) R171.1 R174.1 RD11.2 ; also sheet 1,2,3,5
N$20: K1.3(2:P) RB1.2 RB2.1
N$21: R179.2 R180.2(S) R180.3(E)
N$23: K2.3(2:P) RB2.2 RB3.1
N$26: K3.3(2:P) RB3.2 RB4.1
N$32: K4.3(2:P) RB4.2 RB5.1
N$33: IC32.2(-IN) IC32.6(OUT) R173.1
N$34: IC32.3(+IN) R172.2
N$75: IC33.3(+IN) R175.2
N$76: IC33.2(-IN) IC33.6(OUT) R176.1 R207.2
N$79: K29.3(2:P) R176.2 R177.1
N$80: IC34.2(-IN) K29.4(2:S) R177.2 R179.1
N$85: K5.3(2:P) RB5.2 RB6.1
N$86: K6.3(2:P) RB6.2 RB7.1
N$87: K7.3(2:P) RB7.2 RB8.1
N$88: K8.3(2:P) RB8.2 RB9.1
N$89: K9.3(2:P) RB9.2 RB10.1
N$90: K10.3(2:P) RB10.2 RB11.1
N$91: K1.6(3:P) RA1.2 RA2.1
N$92: K2.6(3:P) RA2.2 RA3.1
N$93: K3.6(3:P) RA3.2 RA4.1
N$94: K4.6(3:P) RA4.2 RA5.1
N$95: K5.6(3:P) RA5.2 RA6.1
N$96: K6.6(3:P) RA6.2 RA7.1
N$97: K7.6(3:P) RA7.2 RA8.1
N$98: K8.6(3:P) RA8.2 RA9.1
N$99: K9.6(3:P) RA9.2 RA10.1
N$100: K10.6(3:P) RA10.2 RA11.1
N$121: CAC1.1 K11.3(2:P)
N$122: CAC2.1 K12.3(2:P)
N$123: CAC3.2 K13.3(2:P)
N$152: CEG1.1 K11.6(3:P)
N$153: CEG2.1 K12.6(3:P)
N$154: CEG3.2 K13.6(3:P)
N$155: CAC4.1 K14.3(2:P)
N$156: CEG4.1 K14.6(3:P)
N$157: K15.3(2:P) RC1.2 RC2.1
N$158: K16.3(2:P) RC2.2 RC3.1
N$159: K17.3(2:P) RC3.2 RC4.1
N$160: K18.3(2:P) RC4.2 RC5.1
N$161: K19.3(2:P) RC5.2 RC6.1
N$162: K20.3(2:P) RC6.2 RC7.1
N$163: K21.3(2:P) RC7.2 RC8.1
N$164: K22.3(2:P) RC8.2 RC9.1
N$165: K23.3(2:P) RC9.2 RC10.1
N$166: K24.3(2:P) RC10.2 RC11.1
N$167: K15.6(3:P) RD1.2 RD2.1
N$168: K16.6(3:P) RD2.2 RD3.1
N$169: K17.6(3:P) RD3.2 RD4.1
N$170: K18.6(3:P) RD4.2 RD5.1
N$171: K19.6(3:P) RD5.2 RD6.1
N$172: K20.6(3:P) RD6.2 RD7.1
N$173: K21.6(3:P) RD7.2 RD8.1
N$174: K22.6(3:P) RD8.2 RD9.1
N$175: K23.6(3:P) RD9.2 RD10.1
N$176: K24.6(3:P) RD10.2 RD11.1
N$177: CBD1.1 K25.3(2:P)
N$178: CBD2.1 K26.3(2:P)
N$179: CBD3.2 K27.3(2:P)
N$180: CDF1.1 K25.6(3:P)
N$181: CDF2.1 K26.6(3:P)
N$182: CDF3.2 K27.6(3:P)
Unconnected: IC32.1(BAL1) IC32.5(BAL2) IC32.8(COMP) IC33.1(BAL1) IC33.5(BAL2) IC33.8(COMP) IC34.1(BAL1) IC34.5(BAL2) IC34.8(COMP) K1.2(2:O) K1.7(3:O) K2.2(2:O) K2.7(3:O) K3.2(2:O) K3.7(3:O) K4.2(2:O) K4.7(3:O) K5.2(2:O) K5.7(3:O) K6.2(2:O) K6.7(3:O) K7.2(2:O) K7.7(3:O) K8.2(2:O) K8.7(3:O) K9.2(2:O) K9.7(3:O) K10.2(2:O) K10.7(3:O) K11.2(2:O) K11.7(3:O) K12.2(2:O) K12.7(3:O) K13.2(2:O) K13.7(3:O) K14.2(2:O) K14.7(3:O) K15.2(2:O) K15.7(3:O) K16.2(2:O) K16.7(3:O) K17.2(2:O) K17.7(3:O) K18.2(2:O) K18.7(3:O) K19.2(2:O) K19.7(3:O) K20.2(2:O) K20.7(3:O) K21.2(2:O) K21.7(3:O) K22.2(2:O) K22.7(3:O) K23.2(2:O) K23.7(3:O) K24.2(2:O) K24.7(3:O) K25.2(2:O) K25.7(3:O) K26.2(2:O) K26.7(3:O) K27.2(2:O) K27.7(3:O) K29.2(2:O)

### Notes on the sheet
- 1K8//4K7 | 1K5//1K5 | 470//4K7 | 390//4K7 | 1K5//1K5
- 1K8//4K7 | 470//4K7 | 390//4K7 | 1K5//1K5
- 1K5//1K5
- 11 | 12
- 1 | 2 | 3 | 4 | 5 | 6 | 7 | 8 | 9 | 10 | 1 | 2 | 3 | 4 | 5 | 6 | 7 | 8 | 9 | 10 | 11
- 20 Hz
- 20 Hz | 25 Hz | 30 Hz | 40 Hz | 50 Hz | 65 Hz | 80 Hz | 100 Hz | 130 Hz | 160 Hz | 200 Hz
- 200 Hz | 2 kHz | 20 kHz | 200 kHz
- 2 kHz | 20 kHz | 200 kHz
- 200 Hz
- 3K9//47K | 2K7//22K | 3K//33K | 2K7//3K9 | 1K//10K | 560//5K6
- 3 | 5 | 7 | 9 | 10 | 11 | 12
- 1 | 2 | 4 | 6 | 8
- 20 Hz
- 200 Hz | 2 kHz
- 20 kHz + 
  200 kHz
- 1 | 2 | 3 | 4 | 5 | 6 | 7 | 8 | 9 | 10 | 11
- DIST.
  CAL.
- 20 Hz | 25 Hz | 30 Hz | 40 Hz | 50 Hz | 65 Hz | 80 Hz | 100 Hz | 130 Hz | 160 Hz | 200 Hz
- PCB3 Sheet 4: Filter Circuits
- S < 0.3 %

## Sheet 5 of 5: Power Supply
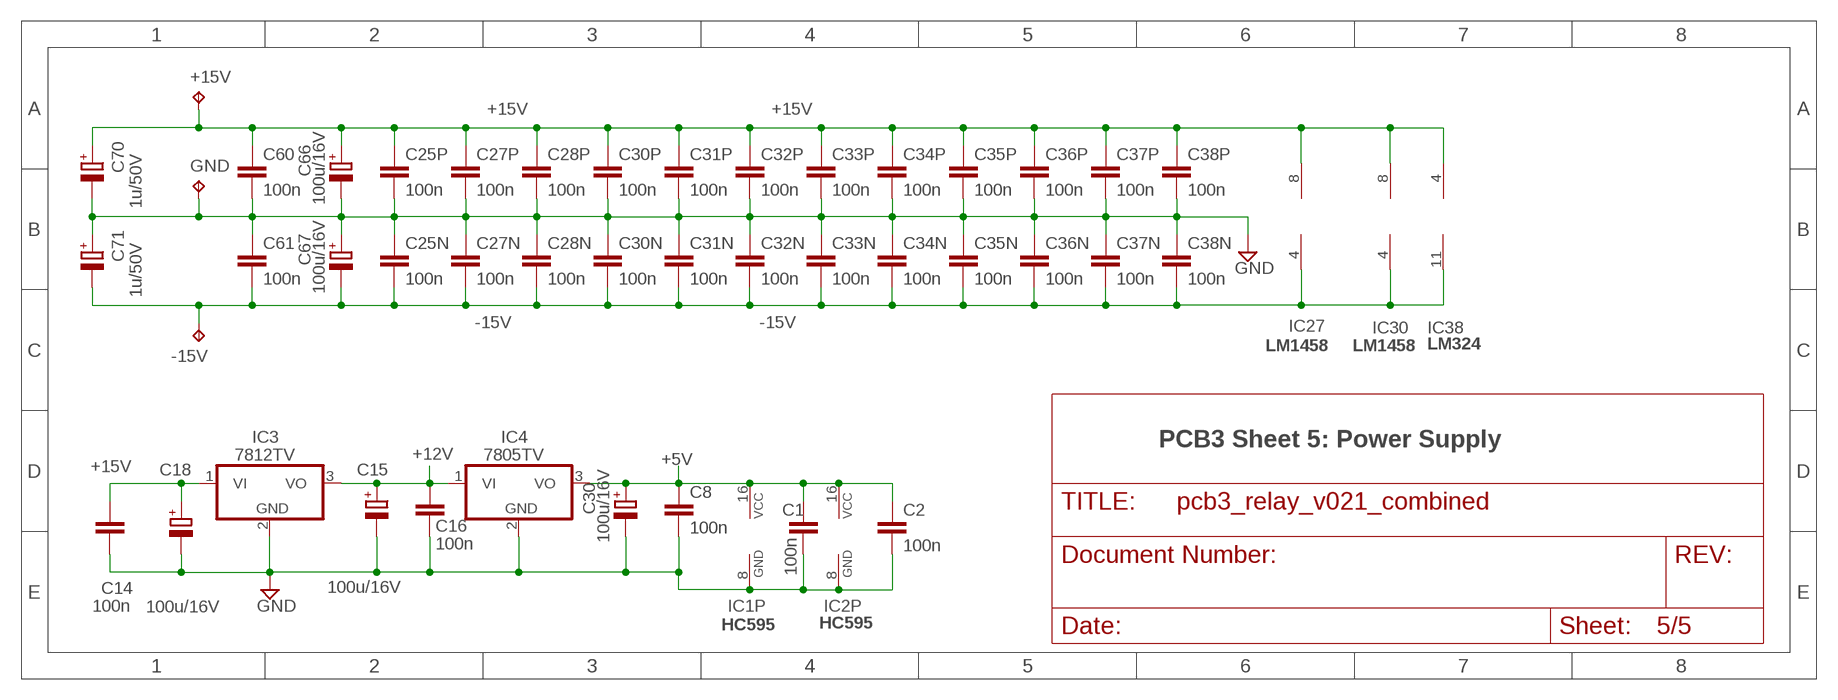
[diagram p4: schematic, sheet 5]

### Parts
+15V  TPPAD1-13Y  [P1-13Y]
-15V  TPPAD1-13Y  [P1-13Y]
C1  100n  C-EUC1206  [C1206]
C2  100n  C-EUC1206  [C1206]
C8  100n  C-EUC1206  [C1206]
C14  100n  C-EUC1206  [C1206]
C15  100u/16V  CPOL-EUUD-6,3X8,8  [UD-6,3X5,8_NICHICON]
C16  100n  C-EUC1206  [C1206]
C18  100u/16V  CPOL-EUUD-6,3X8,8  [UD-6,3X5,8_NICHICON]
C25N  100n  C-EUC1206  [C1206]
C25P  100n  C-EUC1206  [C1206]
C27N  100n  C-EUC1206  [C1206]
C27P  100n  C-EUC1206  [C1206]
C28N  100n  C-EUC1206  [C1206]
C28P  100n  C-EUC1206  [C1206]
C30  100u/16V  CPOL-EUUD-6,3X8,8  [UD-6,3X5,8_NICHICON]
C30N  100n  C-EUC1206  [C1206]
C30P  100n  C-EUC1206  [C1206]
C31N  100n  C-EUC1206  [C1206]
C31P  100n  C-EUC1206  [C1206]
C32N  100n  C-EUC1206  [C1206]
C32P  100n  C-EUC1206  [C1206]
C33N  100n  C-EUC1206  [C1206]
C33P  100n  C-EUC1206  [C1206]
C34N  100n  C-EUC1206  [C1206]
C34P  100n  C-EUC1206  [C1206]
C35N  100n  C-EUC1206  [C1206]
C35P  100n  C-EUC1206  [C1206]
C36N  100n  C-EUC1206  [C1206]
C36P  100n  C-EUC1206  [C1206]
C37N  100n  C-EUC1206  [C1206]
C37P  100n  C-EUC1206  [C1206]
C38N  100n  C-EUC1206  [C1206]
C38P  100n  C-EUC1206  [C1206]
C60  100n  C-EUC1206  [C1206]
C61  100n  C-EUC1206  [C1206]
C66  100u/16V  CPOL-EUUD-6,3X8,8  [UD-6,3X5,8_NICHICON]
C67  100u/16V  CPOL-EUUD-6,3X8,8  [UD-6,3X5,8_NICHICON]
C70  1u/50V  CPOL-EUUD-4X5,8  [UD-4X5,8_NICHICON]
C71  1u/50V  CPOL-EUUD-4X5,8  [UD-4X5,8_NICHICON]
GND  TPPAD1-13Y  [P1-13Y]
IC3  7812TV  [TO220V]
IC4  7805TV  [TO220V]

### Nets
+5V: C1.1 C2.1 C8.1 C30.+ IC1.16(VCC) IC2.16(VCC) IC4.3(VO) ; also sheet 3
+12V: C15.+ C16.1 IC3.3(VO) IC4.1(VI) ; also sheet 3
+15V: +15V.TP C14.1 C18.+ C25P.1 C27P.1 C28P.1 C30P.1 C31P.1 C32P.1 C33P.1 C34P.1 C35P.1 C36P.1 C37P.1 C38P.1 C60.1 C66.+ C70.+ IC3.1(VI) IC27.8(P:V+) IC30.8(P:V+) IC38.4(P:V+) ; also sheet 1,2,4
-15V: -15V.TP C25N.2 C27N.2 C28N.2 C30N.2 C31N.2 C32N.2 C33N.2 C34N.2 C35N.2 C36N.2 C37N.2 C38N.2 C61.2 C67.- C71.- IC27.4(P:V-) IC30.4(P:V-) IC38.11(P:V-) ; also sheet 1,2,4
GND: C1.2 C2.2 C8.2 C14.2 C15.- C16.2 C18.- C25N.1 C25P.2 C27N.1 C27P.2 C28N.1 C28P.2 C30.- C30N.1 C30P.2 C31N.1 C31P.2 C32N.1 C32P.2 C33N.1 C33P.2 C34N.1 C34P.2 C35N.1 C35P.2 C36N.1 C36P.2 C37N.1 C37P.2 C38N.1 C38P.2 C60.2 C61.1 C66.- C67.+ C70.- C71.+ GND.TP IC1.8(GND) IC2.8(GND) IC3.2(GND) IC4.2(GND) ; also sheet 1,2,3,4

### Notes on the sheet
- IC27 | IC30 | IC38
- LM1458 | LM1458 | LM324
- PCB3 Sheet 5: Power Supply
- HC595 | HC595

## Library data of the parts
+15V -15V E21-E23 E29 E31 E32 E37 E40 E42-E47 E49 GND = testpad:TP: Test pad
C1 C2 C8 C14 C16 C25N C25P C27N C27P C28N C28P C30N C30P C31N C31P C32N C32P C33N C33P C34N C34P C35N C35P C36N C36P C37N C37P C38N C38P C54 C58 C60 C61 CAC1-CAC4 CBD1-CBD3 CDF1-CDF3 CEG1-CEG4 = rcl:C-EU: CAPACITOR, European symbol; SPICEPREFIX: C
C15 C18 C30 C52 C53 C55-C57 C59 C66 C67 C70-C74 = rcl:CPOL-EU: POLARIZED CAPACITOR, European symbol; SPICEPREFIX: C
CON1 CON2 = Wurth_Elektronik_Electromechanic_Wire_to_Board_Connectors_rev16a:61200821621: WR-BHD 2.54mm Male Box Header, 8 Pins=>Code : Con_WTB_BHD_2.54_Male_THT_WS_61200821621 Details see: http://katalog.we-online.de/en/em/612_0xx_216_21 Created 2014-06-04, Karrer Zheng 2014 (C) Würth Elektronik
D1 D2 D12-D23 = semicon-smd-ipc:D-: DIODE
DS1-DS29 = diode:DIODE-: DIODE
IC1 IC2 = 74xx-eu:74*595: 8-bit SHIFT REGISTER, output latch
IC3 IC4 = linear:78*: Positive VOLTAGE REGULATOR Source: http://cache.national.com/ds/LM/LM78L05.pdf http://www.fairchildsemi.com/ds/LM/LM7805.pdf
IC25 IC28 = linear:LM318: OP AMP
IC26 IC29 = emile:MC1496
IC27 IC30 = linear:*1458: OP AMP
IC31-IC36 = linear:LM*18: FAST GENERAL-PURPOSE OPERATIONAL AMPLIFIER Sourde: http://focus.ti.com/lit/ds/slos063b/slos063b.pdf
IC37 = linear:*741: OP AMP
IC38 = linear:LM324: OP AMP
K1-K29 = relay:G6K: Low Signal Relay oeiwcsnts1.omron.com/.. D20G6K0100.pdf; MF: OMRON COMPONENTS USA; MPN: G6K-2F-Y DC3; OC_FARNELL: 1690316; OC_NEWARK: 89C6451
QS1-QS29 = semicon-smd-ipc:NPN-TRANSISTOR_: NPN TRANSISTOR
R1 R2 R125-R134 R136-R156 R158-R167 R169-R177 R179 R182-R191 R193-R204 R207 RA1-RA11 RB1-RB11 RC1-RC11 RD1-RD11 = rcl:R-EU_: RESISTOR, European symbol; SPICEPREFIX: R
R135 R157 R180 R192 = rcl:R-TRIMM: Trimm resistor; SPICEMODEL: X; SPICEPREFIXL: POT
RS1-RS29 RS31 = rcl:R-EU_: RESISTOR, European symbol

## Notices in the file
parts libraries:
Wurth_Elektronik_Electromechanic_Wire_to: Copyright: Würth Elektronik
